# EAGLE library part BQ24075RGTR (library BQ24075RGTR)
Standalone 1-cell 1.5-A linear charger, Power Path, 4.2-V VBAT and 5.5-V VOUT 16-VQFN -40 to 85
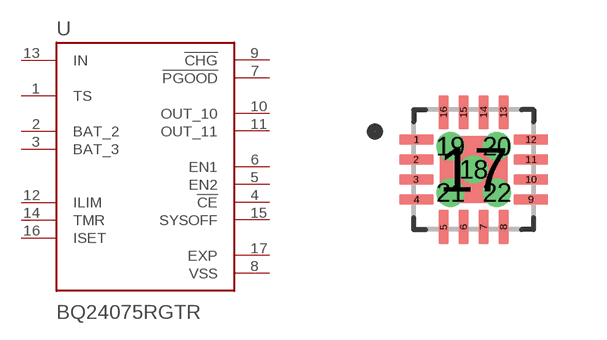
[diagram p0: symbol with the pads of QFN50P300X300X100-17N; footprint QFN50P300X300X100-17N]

Designator prefix U

## BQ24075RGTR (MANUFACTURER: Texas Instruments; MAXIMUM_PACKAGE_HIEGHT: 1mm; PARTREV: M; STANDARD: IPC 7351B)  [QFN50P300X300X100-17N]
1  TS  in
2  BAT_2
3  BAT_3
4  !CE  in
5  EN2  in
6  EN1  in
7  !PGOOD  out
8  VSS  pwr
9  !CHG  out
10  OUT_10  out
11  OUT_11  out
12  ILIM  in
13  IN  in
14  TMR  in
15  SYSOFF  in
16  ISET
17  EXP  pwr

## Footprint QFN50P300X300X100-17N (pad centres in mm)
smd 0.86 x 0.26: 1 -1.435,0.75; 2 -1.435,0.25; 3 -1.435,-0.25; 4 -1.435,-0.75; 9 1.435,-0.75; 10 1.435,-0.25; 11 1.435,0.25; 12 1.435,0.75
smd 0.26 x 0.86: 5 -0.75,-1.435; 6 -0.25,-1.435; 7 0.25,-1.435; 8 0.75,-1.435; 13 0.75,1.435; 14 0.25,1.435; 15 -0.25,1.435; 16 -0.75,1.435
smd 1.68 x 1.68: 17 0,0
drill 0.2 pad 0.4: 18 0,0; 19 -0.58,0.58; 20 0.58,0.58; 21 -0.58,-0.58; 22 0.58,-0.58

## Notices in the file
This work is licensed under a Creative Commons Attribution-ShareAlike 4.0 International License (CC BY-SA) with Design Exception 1.0
